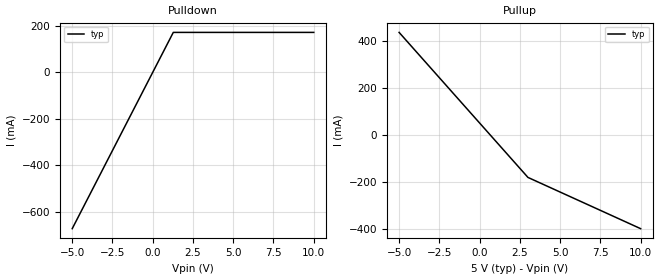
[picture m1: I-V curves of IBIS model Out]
[IBIS Ver]   3.1
[File Name]   bug43.ibs
[File Rev]   0.1
[Component]   TEST
[Manufacturer]   Test File
[Package]
| variable   typ   min   max
R_pkg   0.0m   NA   NA
L_pkg   0.0nH   NA   NA
C_pkg   0.0pF   NA   NA
[Pin]   signal_name   model_name
1   One_Pin   Out
| Models and submodels in the file (1): Out (Output)
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[Model] Out
Model_type Output
Vref=0V
Rref=50ohms
Vmeas=2.5V
|variable   typ  min  max
C_comp   8pF  NA   NA
[Voltage Range]  5V   NA   NA
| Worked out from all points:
|   slope of the pulldown table from 0 to 0.75 V, typ, clamps not added: 7.43 ohm
|   slope of the pullup table from 0 to 0.75 V, typ, clamps not added: 13 ohm
[Pulldown]
|voltage  i(typ)   i(min)  i(max)
-5V       -672.6mA   NA         NA
1.277V    171.8mA    NA         NA
10V       171.8mA    NA         NA
[Pullup]
|voltage  i(typ)   i(min)  i(max)
-5V       437.3mA    NA         NA
3.003V    -179.2mA   NA         NA
10V       -397mA     NA         NA
[Ramp]
|variable  typ   min  max
dV/dt_r   0.0/-851p   -1/0n   0/-1
dV/dt_f   NA   -1/0n   0/-1n
